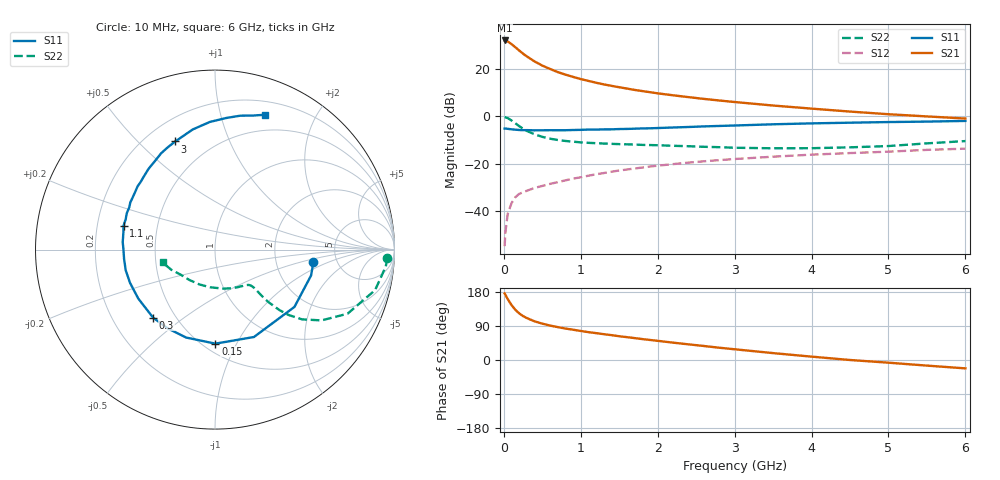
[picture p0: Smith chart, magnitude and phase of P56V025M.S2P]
! SIEMENS Small Signal Semiconductors
! BFP183
! Si NPN RF Bipolar Junction Transistor in SOT143
! VCE = 6 V  IC = 25 mA
! Common Emitter S-Parameters:  March  1996
# GHz  S  MA  R  50
!  f  S11  S21  S12  S22
! GHz  MAG  ANG  MAG  ANG  MAG  ANG  MAG  ANG
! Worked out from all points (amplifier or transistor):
!   36 points, 10 MHz to 6 GHz, reference 50 ohm
!   highest |S21| = 32.1 dB at 10 MHz (marker M1)
!   |S21| within 3 dB of that: start of sweep to 154 MHz
!   unconditionally stable (mu >= 1): 789.3 MHz to 5.715 GHz
!   at 250 MHz: K = 0.51, MSG = 29.3 dB, |S12| = -32.1 dB
!   at 1.4 GHz: K = 1.13, MAG = 16.0 dB, |S12| = -23.4 dB
!   at 6 GHz: K = 0.96, MSG = 6.4 dB, |S12| = -13.6 dB
!   S11 on the Smith chart (normalised r, x): 10 MHz: 3.33, -0.66; 150 MHz: 0.57, -0.82; 300 MHz: 0.38, -0.39; 1.1 GHz: 0.31, +0.12; 3 GHz: 0.32, +0.65; 6 GHz: 0.33, +1.39
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0.01  0.5529 -7.1  40.38 175.6  0.0018 80.9  0.9618 -2.7
0.02  0.5543 -15.1  40.21 172.2  0.0035 80.0  0.956 -5.7
0.05  0.5458 -35.8  38.57 160.8  0.0086 76.8  0.9202 -14.2
0.1  0.5331 -66.0  33.75 144.9  0.0147 64.2  0.8204 -25.8
0.15  0.524 -89.8  28.96 132.4  0.0196 57.6  0.7129 -33.6
0.2  0.5157 -108.2  24.72 123.0  0.023 53.9  0.6216 -38.7
0.25  0.512 -121.1  21.19 115.8  0.0248 51.5  0.549 -41.6
0.3  0.5125 -132.3  18.51 110.6  0.0268 50.4  0.492 -43.2
0.4  0.5071 -147.4  14.54 102.0  0.0307 50.1  0.4173 -44.5
0.5  0.5084 -158.6  11.87 95.9  0.0338 50.3  0.3694 -44.7
0.6  0.5106 -166.9  10.1 90.9  0.0374 51.3  0.3379 -44.5
0.7  0.5093 -174.2  8.658 86.8  0.0406 52.4  0.3171 -44.4
0.8  0.5099 -180.0  7.658 83.0  0.0444 53.0  0.3024 -44.4
1  0.5191 169.5  6.154 76.6  0.0516 53.9  0.2825 -45.1
1.1  0.5266 165.3  5.629 73.5  0.0557 54.0  0.2759 -45.8
1.5  0.5401 150.9  4.133 62.7  0.0718 53.5  0.2592 -50.0
2.2  0.5825 129.5  2.795 45.8  0.0979 48.9  0.2389 -62.7
3  0.6418 110.2  2.015 28.3  0.1254 41.7  0.2172 -82.8
3.5  0.6808 100.5  1.697 18.2  0.1406 37.3  0.2116 -97.7
4.5  0.736 85.1  1.265 0.0  0.1676 28.1  0.2216 -130.4
5.5  0.7761 74.2  0.999 -14.8  0.1959 20.3  0.2689 -155.5
6  0.8022 69.5  0.901 -22.1  0.2078 15.8  0.3008 -166.3
